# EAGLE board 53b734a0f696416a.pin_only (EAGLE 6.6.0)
REV: B

Size 44.45 x 44.2 mm. Coordinates in mm from the lower left corner, seen from the top.
Outline: 0,22.23 arc90 22.23,0 arc90 44.45,22.23 arc80 26.16,44.2 18.29,44.2 arc80 0,22.23
Copper layers (1*16): Top 0.035mm / dielectric 1.5mm / Bottom 0.035mm
Design rules "adafruit": minimum track width 8mil, minimum drill 15.5mil, track to track 8mil, track to pad 8mil, pad to pad 8mil, via to via 8mil, smd to smd 8mil, copper to edge 10mil, drill to drill 8mil, minimum pad ring 10mil, minimum via ring 8mil, stop-mask expansion 2mil, vias tented up to drill 20mil, thermal gap 10mil

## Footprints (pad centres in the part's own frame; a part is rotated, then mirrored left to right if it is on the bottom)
SEWINGTAP_2.0 = drill 1.5 pad 2.54: P$1 0,0
JST-PH-2-SMT-RA = smd 1 x 4.6: 1 1,-3.7; 2 -1,-3.7 | smd 1.6 x 3.4: NC1 -3.4,1.5; NC2 3.4,1.5
KMR2 = smd 1 x 1: 1 2,0.8; 2 2,-0.8; 3 -2,0.8; 4 -2,-0.8
0805-NO = smd 1.3 x 1.5: 1 -0.95,0; 2 0.95,0
_0805MP = smd 1.2 x 1.3: 1 -1.016,0; 2 1.016,0
4UCONN_20329 = smd 1 x 2: BASE@1 -0.75,-2; BASE@2 0.75,-2 | smd 0.4 x 1.35: D+ 0,0.775; D- -0.65,0.775; GND 1.3,0.775; ID 0.65,0.775; VBUS -1.3,0.775 | drill 0.7 offset: SPRT@1 -3.3,0.9; SPRT@2 3.3,0.9 | drill 0.6 pad 2.5 square: SPRT@3 -3.6,-1.9; SPRT@4 3.6,-1.9 | hole 0.7: -1.95,0; 1.95,0
SOD-123 = smd 1.4 x 1.4: A 1.85,0; C -1.85,0
TQFP44 = smd 1.5 x 0.5: 1 -5.8,4; 2 -5.8,3.2; 3 -5.8,2.4; 4 -5.8,1.6; 5 -5.8,0.8; 6 -5.8,0; 7 -5.8,-0.8; 8 -5.8,-1.6; 9 -5.8,-2.4; 10 -5.8,-3.2; 11 -5.8,-4; 23 5.8,-4; 24 5.8,-3.2; 25 5.8,-2.4; 26 5.8,-1.6; 27 5.8,-0.8; 28 5.8,0; 29 5.8,0.8; 30 5.8,1.6; 31 5.8,2.4; 32 5.8,3.2; 33 5.8,4 | smd 0.5 x 1.5: 12 -4,-5.8; 13 -3.2,-5.8; 14 -2.4,-5.8; 15 -1.6,-5.8; 16 -0.8,-5.8; 17 0,-5.8; 18 0.8,-5.8; 19 1.6,-5.8; 20 2.4,-5.8; 21 3.2,-5.8; 22 4,-5.8; 34 4,5.8; 35 3.2,5.8; 36 2.4,5.8; 37 1.6,5.8; 38 0.8,5.8; 39 0,5.8; 40 -0.8,5.8; 41 -1.6,5.8; 42 -2.4,5.8; 43 -3.2,5.8; 44 -4,5.8
SOT23-5L = smd 0.55 x 1.2: 1 -0.95,-1.3; 2 0,-1.3; 3 0.95,-1.3; 4 0.95,1.3; 5 -0.95,1.3
2X03 = drill 1.016 octagon: 1 -2.54,-1.27; 2 -2.54,1.27; 3 0,-1.27; 4 0,1.27; 5 2.54,-1.27; 6 2.54,1.27
CHIPLED_0805_NOOUTLINE = smd 1.2 x 1.2: A 0,-1.05; C 0,1.05
R1206 = smd 1.6 x 1.803: 1 -1.422,0; 2 1.422,0
WS2812 = smd 2 x 1.1: DI 2,0; DO 2,-1.7; LEDVDD -2,0; NC -2,1.7; VDD 2,1.7; VSS -2,-1.7
EG1390 = smd 1 x 1.5: O1 -2.5,2.8; O2 -2.5,-2.8; P1 0,2.8; P2 0,-2.8; S1 2.5,2.8; S2 2.5,-2.8 | hole 1: 1.5,0; -1.5,0
SOT-23 = smd 0.787 x 0.889: 1 0.025,-1.016; 2 -0.94,1.016; 3 0.991,1.016
FIDUCIAL_1MM = smd 1 x 1: 1 0,0
RESONATOR-SMD = smd 0.7 x 1.7: 1 -1.2,0; 2 0,0; 3 1.2,0

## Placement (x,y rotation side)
3.3VTAP  SEWTAP-2.0IN  [SEWINGTAP_2.0]  2.67,22.23 90 top
3V3TAP2  SEWTAP-2.0IN  [SEWINGTAP_2.0]  32.13,39.24 330 top
BATT  3-9VDC  [JST-PH-2-SMT-RA]  22.23,3.68 180 top
BOOT  SPST_TACT-KMR2  [KMR2]  22.23,12.07 180 top
C4  10uF  [0805-NO]  34.42,14.35 90 top
C5  10uF  [0805-NO]  32.13,10.92 0 top
C6  10uF  [0805-NO]  32.64,32.26 270 top
C7  10uF  [0805-NO]  30.35,17.91 90 top
C8  10uF  [0805-NO]  14.99,9.65 180 top
C9  10uF  [_0805MP]  19.43,35.81 90 top
CN1  MiniB USB  [4UCONN_20329]  22.23,39.88 180 top
D1  SCHOTTKY  [SOD-123]  32.77,28.58 180 top
D2  SCHOTTKY  [SOD-123]  27.56,9.78 180 top
D6  SEWTAP-2.0IN  [SEWINGTAP_2.0]  40.77,15.62 250 top
GND3TAP  SEWTAP-2.0IN  [SEWINGTAP_2.0]  12.32,39.24 30 top
GNDTAP  SEWTAP-2.0IN  [SEWINGTAP_2.0]  41.78,22.23 270 top
GNDTAP2  SEWTAP-2.0IN  [SEWINGTAP_2.0]  12.32,5.21 150 top
IC1  ATMEGA32U4-AU  [TQFP44]  22.23,26.16 270 top
IC2  MIC5225-3.3V  [SOT23-5L]  31.24,14.1 270 top
IO9  SEWTAP-2.0IN  [SEWINGTAP_2.0]  40.77,28.83 290 top
IO10  SEWTAP-2.0IN  [SEWINGTAP_2.0]  37.21,34.92 310 top
IO12  SEWTAP-2.0IN  [SEWINGTAP_2.0]  37.21,9.53 230 top
JP1  ICSP  [2X03]  34.16,20.32 90 top
L  RED  [CHIPLED_0805_NOOUTLINE]  29.21,34.54 180 top
L1  500mA  [R1206]  27.43,35.18 270 top
LED1  WS2812  [WS2812]  22.23,16.51 0 top
ON/OFF  EG1390  [EG1390]  10.41,22.23 90 top
PWR  GREEN  [CHIPLED_0805_NOOUTLINE]  15.24,34.67 180 top
R1  22  [0805-NO]  25.02,35.94 270 top
R2  22  [0805-NO]  23.11,35.81 270 top
R3  1K  [_0805MP]  21.21,35.81 270 top
R4  1K  [_0805MP]  17.53,35.81 90 top
R5  1K  [0805-NO]  29.97,31.5 0 top
R6  1K  [0805-NO]  9.53,29.72 90 top
R7  10K  [_0805MP]  12.32,16.64 270 top
R8  150K  [0805-NO]  30.48,25.91 270 top
R9  10K  [0805-NO]  33.27,25.65 0 top
R10  2.2K  [0805-NO]  26.67,17.27 90 top
RX  SEWTAP-2.0IN  [SEWINGTAP_2.0]  3.68,15.62 110 top
RXLED  YELLOW  [CHIPLED_0805_NOOUTLINE]  11.56,29.72 0 top
SCL  SEWTAP-2.0IN  [SEWINGTAP_2.0]  7.24,34.92 50 top
SDA  SEWTAP-2.0IN  [SEWINGTAP_2.0]  3.68,28.83 70 top
T1  DMG3415  [SOT-23]  27.56,12.45 180 top
TX  SEWTAP-2.0IN  [SEWINGTAP_2.0]  7.24,9.53 130 top
TXLED  YELLOW  [CHIPLED_0805_NOOUTLINE]  13.34,29.72 0 top
U$1  [ADAFRUIT_5MM]  13.59,11.43 0 top
U$2  FIDUCIAL""  [FIDUCIAL_1MM]  12.07,10.8 0 top
U$3  FIDUCIAL""  [FIDUCIAL_1MM]  11.94,33.91 0 top
U$4  [FLORAMED]  33.91,24.13 0 bottom
U$5  [PCBFEAT-REV-040]  21.59,8.89 0 bottom
U$6  FIDUCIAL""  [FIDUCIAL_1MM]  35.18,30.86 0 top
U$7  [SYMBOL_FCC_5MM]  28.7,2.29 0 bottom
U$8  [SYMBOL_CE_5MM]  20.57,2.41 0 bottom
VCC2  SEWTAP-2.0IN  [SEWINGTAP_2.0]  32.13,5.21 210 top
Y1  8MHz  [RESONATOR-SMD]  16.13,19.3 90 top

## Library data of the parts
3.3VTAP 3V3TAP2 BATT BOOT D6 GND3TAP GNDTAP GNDTAP2 IC2 IO9 IO10 IO12 L1 LED1 ON/OFF RX SCL SDA TX VCC2 = adafruit
C4-C9 CN1 D1 D2 L PWR R1-R10 RXLED TXLED U$1 U$5 U$7 U$8 = microbuilder
IC1 = adaprog
JP1 = pinhead
T1 = zetex; OC_FARNELL: unknown; OC_NEWARK: unknown
U$2 U$3 U$6 = microbuilder; BOM: EXCLUDE
U$4 = flora
Y1 = SparkFun

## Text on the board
tPlace: GND | 3.3V | SCL | D7 | PWR | adafruit! | D10 | RX | TX | SDA | D9 | OFF | 3.3V | GND | D6 | RX | ON | D12 | TX | VBATT | GND
bPlace: Mainboard version B | Atmega32u4 @ 8 MHz | VBatt: 3-9VDC

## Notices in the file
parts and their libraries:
microbuilder: This work is placed in the public domain, and may be freely used for commercial and non-commercial work with the following conditions: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
SparkFun: Licensing: CC v3.0 Share-Alike You are welcome to use this library for commercial purposes.
